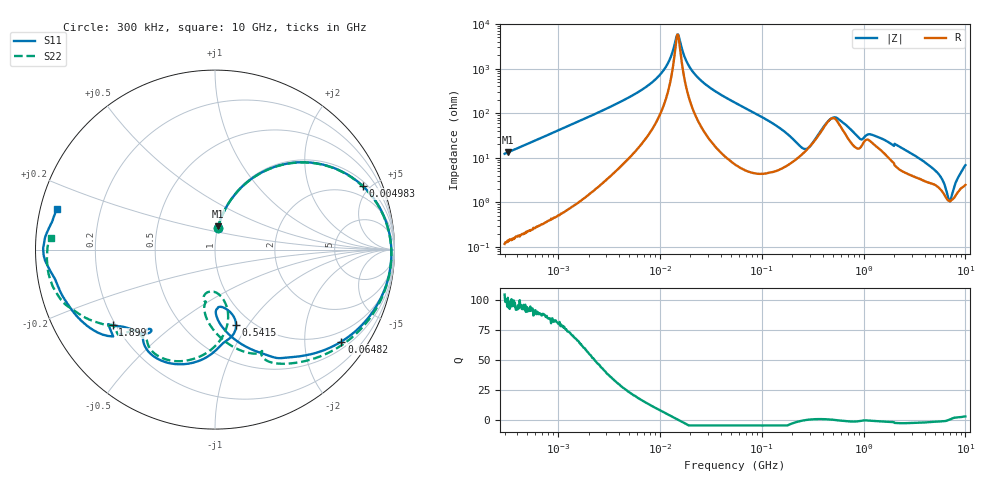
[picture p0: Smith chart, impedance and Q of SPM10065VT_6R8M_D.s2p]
! S-Parameter Data Generated by TDK Corporation
! Copyright(C) 2020 TDK Corporation.
! All Rights Reserved.
! TDK P/N: SPM10065VT-6R8M-D (Inductor)
! Property: L=6.8uH at 100kHz
! Size(LxWxT): 10.5x10x6.5mm
! Model Type: s2p (Touchstone File Format Version 1.0)
! Frequency: DC=Yes Start=0.3MHz Stop=10000MHz 802points Log-sweep
! Model Generated on Apr. 23, 2020
! Port Assignments:
!  1 ---@@@--- 2
! Applicable Conditions:
!  Temperature = 25 degC
!  DC Bias Current = 0 A
!  Small Signal Operation
! Terms and conditions regarding TDK Simulation Models
! (1)This simulation model is being provided solely for informational purposes. Please refer to the specifications of the products in terms of detailed characteristics of such products.
! (2)In no event shall TDK Corporation of any of its subsidiaries be liable for any loss or damage arising, directly or indirectly,
!  From any information contained in this simulation model, including, but not limited to loss or damages arising from any inaccuracies, omissions or errors in connection with such information.
! (3)Any and all copyrights on this simulation model are owned by TDK Corporation.
!  Duplication or redistribution of this simulation model without prior written permission from TDK Corporation is prohibited.
! (4)This simulation model is subject to any modification or change without any prior notice.
! (5)Neither TDK Corporation nor any of its subsidiaries shall make any warranty, express or implied,
!  Including but not limited to the correctness, implied warranties of merchantability and fitness for a particular purpose with respect to this simulation models.
! (6)The use of this simulation model shall be deemed to have consented to the terms and conditions hereof.
# Hz S MA R 50
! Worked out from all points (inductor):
!   801 points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, 300 kHz to 10 GHz, reference 50 ohm
!   read as 1/Y11, port 2 shorted: L = 6.51 uH near 318.3 kHz
!   highest Q = 101 at 322.9 kHz (marker M1), where L = 6.53 uH
!   self-resonance near 14.9 MHz
!   S11 on the Smith chart (normalised r, x): 300 kHz: 1.00, +0.25; 4.983 MHz: 1.25, +4.51; 64.82 MHz: 0.69, -2.93; 541.5 MHz: 0.85, -0.88; 1.899 GHz: 0.19, -0.32; 10 GHz: 0.05, +0.13
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300000  0.1228 82.7  0.9907 -7.0  0.991 -7.0  0.1227 82.6
322921  0.1318 82.2  0.9895 -7.5  0.9898 -7.5  0.1318 82.0
1713600  0.5695 54.1  0.813 -35.0  0.8128 -35.0  0.5696 54.0
4982740  0.8959 23.3  0.4081 -64.4  0.408 -64.4  0.8961 23.1
9671944  0.9685 8.3  0.17 -76.2  0.1699 -76.2  0.9685 7.8
1.322782e7  0.9804 2.3  0.07552 -75.4  0.07551 -75.4  0.9805 1.6
1.717743e7  0.9833 -2.6  0.0164 3.9  0.01639 3.9  0.9835 -3.5
2.063197e7  0.9819 -6.1  0.05737 66.9  0.05734 66.9  0.9819 -7.2
2.53611e7  0.9765 -10.3  0.1176 71.1  0.1176 71.1  0.9766 -11.7
5.477226e7  0.9035 -30.4  0.384 55.2  0.3838 55.2  0.903 -33.4
6.481723e7  0.8707 -36.1  0.4505 49.4  0.4503 49.4  0.8697 -39.6
1.720721e8  0.5457 -74.4  0.7671 4.6  0.7668 4.6  0.5362 -81.2
3.126428e8  0.3631 -89.0  0.7696 -32.2  0.7694 -32.2  0.3391 -100.1
4.20949e8  0.32 -85.7  0.667 -55.3  0.6668 -55.3  0.2946 -99.9
5.414944e8  0.4381 -74.4  0.4659 -69.2  0.4657 -69.2  0.2519 -102.3
6.904357e8  0.6083 -95.4  0.3578 -78.2  0.3576 -78.2  0.4284 -81.0
8.758105e8  0.6852 -120.4  0.3095 -71.5  0.3093 -71.5  0.639 -104.5
1.117505e9  0.5874 -128.1  0.3713 -92.1  0.3711 -92.1  0.6326 -127.0
1.767019e9  0.6847 -141.5  0.235 -143.9  0.2349 -143.8  0.672 -136.7
1.898818e9  0.7089 -143.5  0.2081 -153.6  0.2079 -153.6  0.7 -137.9
5.099159e9  0.9072 -169.7  0.0125 151.8  0.01248 151.9  0.9159 -164.8
1e10  0.9075 165.5  0.01317 137.5  0.01312 138.0  0.9175 176.1
